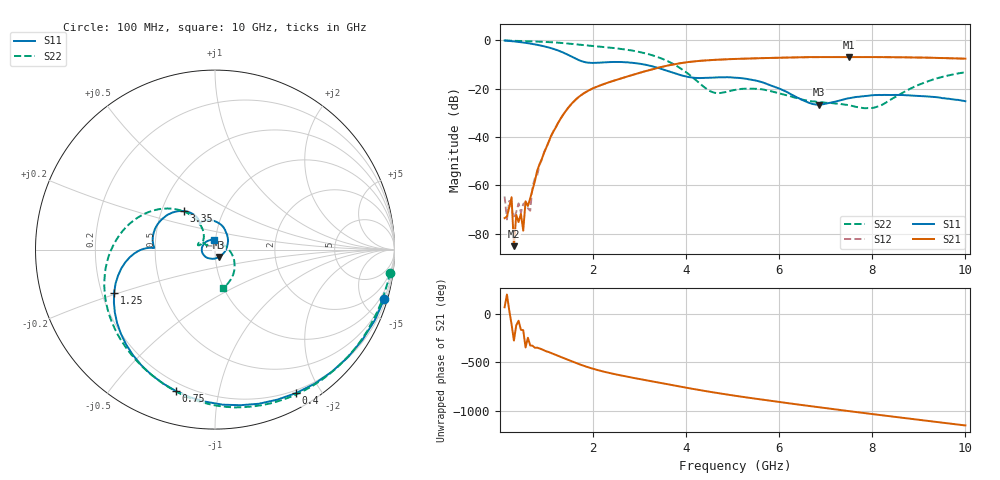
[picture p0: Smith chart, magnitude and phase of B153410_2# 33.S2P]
!  2-Port S-parameters saved by WinCal
! VAR MeasName=S-Parameters (CALIBRATED_DATA) read from VNA (N5245A)
! VAR MeasDate=2016-12-23 10:01:04
! VAR NAME=B153410_2# 33
! VAR FILENAME=B153410_2# 33.S2P
! VAR DATE=2016-12-23 10:01:04
! VAR PHYS_PORTS=1,2
# Hz S DB R 50
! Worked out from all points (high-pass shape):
!   199 points, 100 MHz to 10 GHz, reference 50 ohm
!   highest |S21| = -6.95 dB at 7.5 GHz (marker M1); lowest = -85.1 dB at 300 MHz (marker M2)
!   |S21| within 3 dB of the highest: 3.75 GHz to end of sweep
!   lowest |S11| = -26.7 dB at 6.85 GHz (marker M3), VSWR 1.10, Z = 52.1 - j4.25 ohm
!   |S11| at or under -10 dB: 3.081 GHz to end of sweep
!   |S22| runs from -28.1 to -0.1 dB; largest |S21 - S12| = 0.0029
!   S11 on the Smith chart (normalised r, x): 100 MHz: 0.44, -7.01; 400 MHz: 0.17, -1.70; 750 MHz: 0.16, -0.75; 1.25 GHz: 0.25, -0.19; 3.35 GHz: 0.65, +0.30; 10 GHz: 0.98, +0.11
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1e8  -0.15 -16.2  -73.50 70.5  -64.53 -84.7  -0.14 -7.5
1.5e8  -0.23 -23.9  -72.87 -158.4  -74.07 46.4  -0.18 -10.9
2e8  -0.33 -31.5  -69.02 36.4  -66.40 -51.6  -0.22 -14.3
2.5e8  -0.42 -39.0  -64.87 -107.0  -69.43 -68.6  -0.25 -17.6
3e8  -0.52 -46.3  -85.10 86.5  -73.70 -149.6  -0.28 -21.0
3.5e8  -0.62 -53.5  -72.17 -116.1  -71.03 -82.7  -0.32 -24.3
4e8  -0.74 -60.5  -75.13 -68.6  -67.42 -93.5  -0.33 -27.6
4.5e8  -0.86 -67.4  -71.73 -161.6  -71.31 -34.2  -0.36 -30.9
5e8  -0.98 -74.1  -78.69 -166.8  -67.68 39.6  -0.39 -34.2
5.5e8  -1.13 -80.7  -66.54 15.1  -67.03 44.6  -0.42 -37.5
6.5e8  -1.42 -93.4  -65.36 36.2  -70.49 40.9  -0.49 -44.1
7.5e8  -1.75 -105.5  -58.33 12.1  -57.08 27.0  -0.55 -50.6
1.25e9  -4.28 -156.9  -34.18 -72.0  -34.15 -71.7  -1.05 -82.8
1.75e9  -8.67 178.5  -22.67 -165.8  -22.61 -165.7  -1.98 -112.5
3.35e9  -11.21 128.8  -11.66 17.6  -11.65 17.5  -6.73 156.5
3.4e9  -11.48 127.1  -11.42 13.2  -11.41 13.0  -7.08 153.5
5.05e9  -15.47 102.9  -7.77 -123.5  -7.79 -123.4  -20.56 165.5
6.7e9  -26.28 -36.1  -7.00 127.1  -7.01 127.2  -25.27 153.1
6.85e9  -26.66 -60.9  -6.99 117.7  -6.99 117.6  -25.54 154.1
7.5e9  -23.99 -134.2  -6.95 77.6  -6.96 77.5  -26.86 132.7
8.35e9  -22.65 -178.0  -7.07 26.6  -7.04 26.5  -25.09 25.0
1e10  -25.23 97.2  -7.65 -70.3  -7.69 -70.2  -13.26 -77.7
